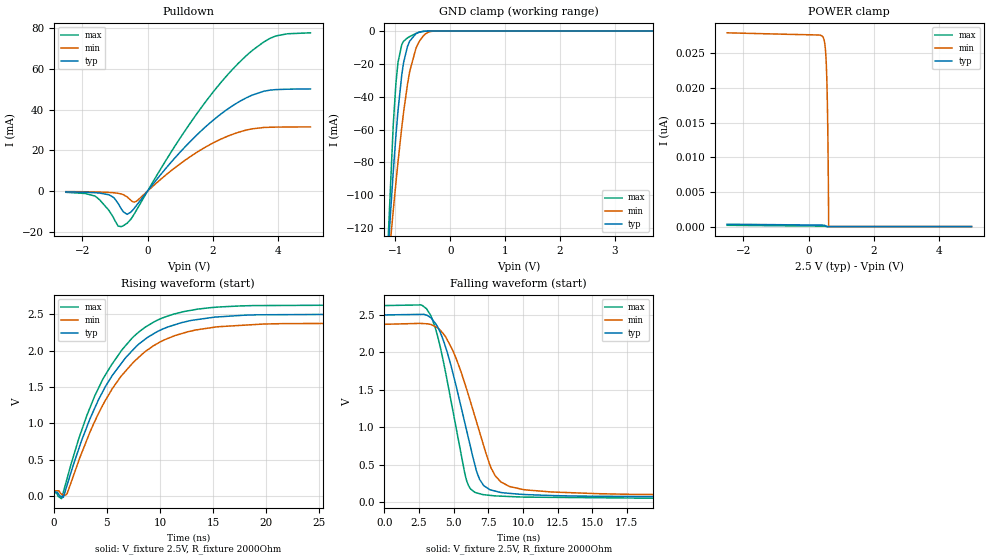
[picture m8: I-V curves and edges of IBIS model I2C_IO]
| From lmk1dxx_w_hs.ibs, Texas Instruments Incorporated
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|   I2C_IO Model
[Model]   I2C_IO
Model_type   I/O_open_drain
Polarity   Non-Inverting
Enable   Active-Low
Vinl = 0.75
Vinh = 1.75
Vmeas = 1.25
Vref = 2.5
Cref = 2pF
Rref = 2000
|   typ   min   max
C_comp   2.068pF   1.93pF   2.196pF
[Voltage Range]   2.5   2.375   2.625
[Temperature Range]   45   150   -40
[Pullup Reference]   2.5   2.375   2.625
[Pulldown Reference]   0   0   0
[Power Clamp Reference]   2.5   2.375   2.625
[GND Clamp Reference]   0   0   0
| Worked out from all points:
|   slope of the pulldown table from 0 to 0.375 V, typ, clamps not added: 49.6 ohm
|   GND clamp passes 1 mA (typ) near -0.58 V on its own axis
|   falling waveform, V_fixture 2.5V, R_fixture 2000Ohm: 20-80 % time 1.95ns typ, 2.36ns min, 1.64ns max; typ from 2.5 V to 0.06 V
|   rising waveform, V_fixture 2.5V, R_fixture 2000Ohm: 20-80 % time 5.37ns typ, 5.6ns min, 5.14ns max; typ from 0.06 V to 2.5 V
[Pulldown]
|   Voltage   I(typ)   I(min)   I(max)
-2.5V     -354.9uA   -215.8uA   -574.4uA
-1.582V   -816.2uA   -398.3uA   -2.753mA
-1.058V   -2.92mA    -774.1uA   -12.6mA
-900.2mV  -6.075mA   -1.079mA   -17.18mA
-740.5mV  -10.21mA   -1.755mA   -16.95mA
-625mV    -11.37mA   -2.828mA   -15.74mA
-357.3mV  -7.414mA   -5.11mA    -9.847mA
1.292V    24.03mA    16.71mA    32.93mA
2.038V    35.11mA    23.86mA    49.12mA
2.741V    43.21mA    28.62mA    61.97mA
3.763V    49.58mA    31.36mA    75.01mA
5V        50.18mA    31.54mA    77.7mA
[GND Clamp]
|   Voltage   I(typ)   I(min)   I(max)
-2.5V     -1.007A    -724.9mA   -1.655A
-1.123V   -128.8mA   -140.3mA   -120.6mA
-1.038V   -85.77mA   -109.3mA   -57.26mA
-989.5mV  -63.72mA   -92.39mA   -31.86mA
-951.3mV  -48.39mA   -79.7mA    -19.04mA
-883mV    -26.76mA   -58.72mA   -8.31mA
-848.5mV  -19.05mA   -49.12mA   -6.18mA
-738.2mV  -6.13mA    -24.62mA   -3.381mA
-625mV    -1.656mA   -10.63mA   -1.469mA
-480.3mV  -197.7uA   -2.675mA   -152uA
-305.5mV  -7.07uA    -89.1uA    -5.456uA
5V        0A         0A         0A
[POWER Clamp]
|   Voltage   I(typ)   I(min)   I(max)
-2.5V     340.6pA    27.93nA    186.5pA
440.7mV   210.8pA    27.32nA    68.72pA
483.5mV   185.4pA    26.72nA    65.97pA
514.2mV   125.4pA    25.63nA    60.89pA
537.5mV   13.32pA    23.98nA    50.55pA
554mV     0A         22.04nA    34.26pA
570.5mV   0A         19.07nA    0A
587.7mV   0A         14.31nA    0A
601.2mV   0A         8.839nA    0A
616.2mV   0A         155.4pA    0A
617.8mV   0A         0A         0A
5V        0A         0A         0A
[Ramp]
R_load = 2000
|   typ   min   max
dV/dt_r   1.46428/5.34885e-09   1.37809/5.56794e-09   1.54667/5.11923e-09
dV/dt_f   1.46428/1.94117e-09   1.37809/2.34844e-09   1.54667/1.62746e-09
[Falling Waveform]
V_fixture = 2.5V
V_fixture_min = 2.375V
V_fixture_max = 2.625V
R_fixture = 2000Ohm
C_fixture = 0F
|   Time   V(typ)   V(min)   V(max)
0s        2.5V       2.375V     2.625V
3.04ns    2.497V     2.382V     2.583V
3.701ns   2.383V     2.343V     2.311V
4.297ns   2.14V      2.24V      1.844V
6.071ns   852.4mV    1.43V      223.3mV
6.87ns    305.6mV    937.2mV    113.8mV
7.984ns   149.5mV    356.6mV    84.96mV
9.701ns   107.5mV    182.3mV    70.8mV
62.28ns   60.66mV    79.78mV    48.15mV
500ns     59.53mV    78.14mV    47.21mV
[Rising Waveform]
V_fixture = 2.5V
V_fixture_min = 2.375V
V_fixture_max = 2.625V
R_fixture = 2000Ohm
C_fixture = 0F
|   Time   V(typ)   V(min)   V(max)
0s        59.53mV    78.14mV    47.21mV
728.4ps   -2.363mV   32.06mV    -30.52mV
1.249ns   155.6mV    40.66mV    246.3mV
2.406ns   677mV      513.8mV    816.4mV
3.856ns   1.212V     1.029V     1.379V
5.511ns   1.659V     1.479V     1.819V
7.336ns   1.991V     1.813V     2.165V
11.42ns   2.354V     2.206V     2.503V
17.55ns   2.48V      2.344V     2.611V
500ns     2.5V       2.375V     2.625V
